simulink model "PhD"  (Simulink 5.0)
settings: Solver=ode4  StartTime=0.0  StopTime=10  FixedStep=0.01  RelTol=1e-3
libraries: simulink x1

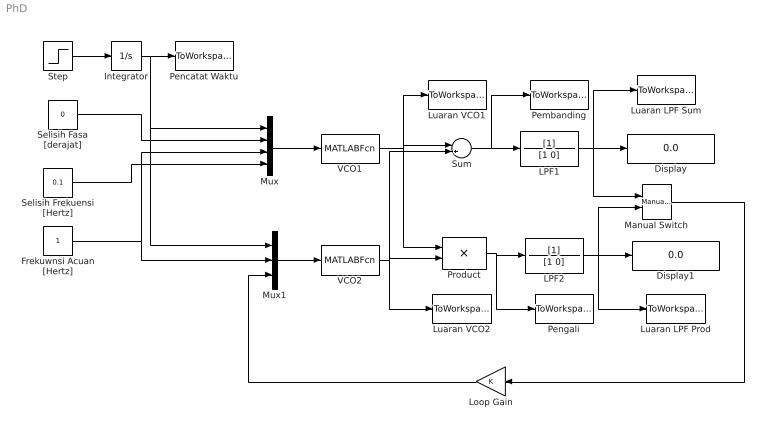
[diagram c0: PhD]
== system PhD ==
  Display : Display
  Display1 : Display
  Frekuwnsi Acuan [Hertz] : Constant
  Integrator : Integrator
  LPF1 : TransferFcn  Denominator=[1 0]
  LPF2 : TransferFcn  Denominator=[1 0]
  Loop Gain : Gain  Orientation=left
  Luaran LPF Prod : ToWorkspace  VariableName=voutprod  SampleTime=-1  SaveFormat=Array
  Luaran LPF Sum : ToWorkspace  VariableName=voutsum  SampleTime=-1  SaveFormat=Array
  Luaran VCO1 : ToWorkspace  VariableName=outvco1  SampleTime=-1  SaveFormat=Array
  Luaran VCO2 : ToWorkspace  VariableName=outvco2  SampleTime=-1  SaveFormat=Array
  Manual Switch : simulink/Signal Routing/Manual Switch  sw=1  action=0
  Mux : Mux
  Mux1 : Mux  Inputs=3
  Pembanding : ToWorkspace  VariableName=outsum  SampleTime=-1  SaveFormat=Array
  Pencatat Waktu : ToWorkspace  VariableName=time  SampleTime=-1  SaveFormat=Array
  Pengali : ToWorkspace  VariableName=outprod  SampleTime=-1  SaveFormat=Array
  Product : Product
  Selisih Fasa [derajat] : Constant  Value=0
  Selisih Frekuensi [Hertz] : Constant  Value=0.1
  Step : Step  Time=0  SampleTime=0
  Sum : Sum  Inputs=|+-
  VCO1 : MATLABFcn  MATLABFcn=vco1
  VCO2 : MATLABFcn  MATLABFcn=vco2
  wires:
  Step/1 -> Integrator/1
  Integrator/1 -> Pencatat Waktu/1, Mux/1, Mux1/1
  Frekuwnsi Acuan [Hertz]/1 -> Mux1/2, Mux/3
  Selisih Fasa [derajat]/1 -> Mux/2
  Selisih Frekuensi [Hertz]/1 -> Mux/4
  Mux/1 -> VCO1/1
  Mux1/1 -> VCO2/1
  VCO1/1 -> Sum/1, Product/1, Luaran VCO1/1
  VCO2/1 -> Sum/2, Product/2, Luaran VCO2/1
  Sum/1 -> LPF1/1, Pembanding/1
  Product/1 -> LPF2/1, Pengali/1
  LPF1/1 -> Display/1, Luaran LPF Sum/1, Manual Switch/1
  LPF2/1 -> Display1/1, Luaran LPF Prod/1, Manual Switch/2
  Manual Switch/1 -> Loop Gain/1
  Loop Gain/1 -> Mux1/3
